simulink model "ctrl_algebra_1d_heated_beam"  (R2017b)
settings: Solver=ode45  StartTime=0.0  StopTime=4000  RelTol=1e-3
undefined symbols (not defined in the file or in its folder): b
libraries: dps x8

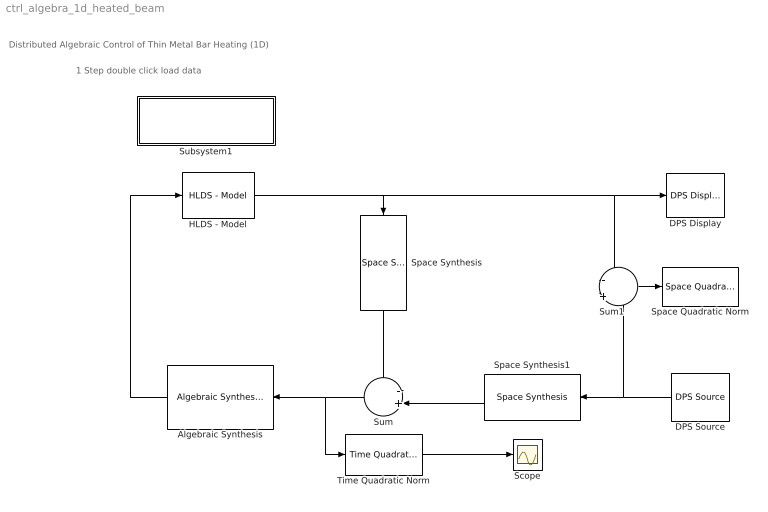
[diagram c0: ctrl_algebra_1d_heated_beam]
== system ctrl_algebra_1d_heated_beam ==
  note: Distributed Algebraic Control of Thin Metal Bar Heating (1D)
  note: 1 Step double click load data
  Algebraic Synthesis : dps/Temporal Synthesis/Algebraic Synthesis  kriterium=deadbeat  b=b  a=a  samplePeriod=40
  DPS Display : dps/DPS Display  graphType=surf  pointCoord=[0:10]'  elementsVar=[1 2; 2 3; 3 4; 4 5; 5 6; 6 7; 7 8; 8 9; 9 10; 10 11]  showColor=on  minC=0  maxC=200  showDeform=off  deform=z  deformScale=0.001  showScope=off  responseVar=H  aviparam=0
  DPS Source : dps/DPS Source  equation='readW(t)'  responseVar=0  showInput=on  pointsCoord=[0:10]'  elementsVar=[1 2; 2 3; 3 4; 4 5; 5 6; 6 7; 7 8; 8 9; 9 10; 10 11]  samplePeriod=40
  HLDS - Model : dps/Controlled Systems/HLDS - Model  StepResponse=H  samplePeriod=40  u_step=1
  Scope : Scope
  Space Quadratic Norm : dps/Quadratic norms/Space Quadratic Norm  StepResponse=H  showNorm=on
  Space Synthesis : dps/Space Synthesis/Space Synthesis  PCH=H  weights=[]
  Space Synthesis1 : dps/Space Synthesis/Space Synthesis  PCH=H  weights=[]
  Subsystem1 : Subsystem
  Sum : Sum  Inputs=-+|
  Sum1 : Sum  Inputs=-|+
  Time Quadratic Norm : dps/Quadratic norms/Time Quadratic Norm
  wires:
  Algebraic Synthesis/1 -> HLDS - Model/1
  HLDS - Model/1 -> Space Synthesis/1, Sum1/1, DPS Display/1
  Sum/1 -> Time Quadratic Norm/1, Algebraic Synthesis/1
  Space Synthesis/1 -> Sum/1
  DPS Source/1 -> Sum1/2, Space Synthesis1/1
  Space Synthesis1/1 -> Sum/2
  Time Quadratic Norm/1 -> Scope/1
  Sum1/1 -> Space Quadratic Norm/1

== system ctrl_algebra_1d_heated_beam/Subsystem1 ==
